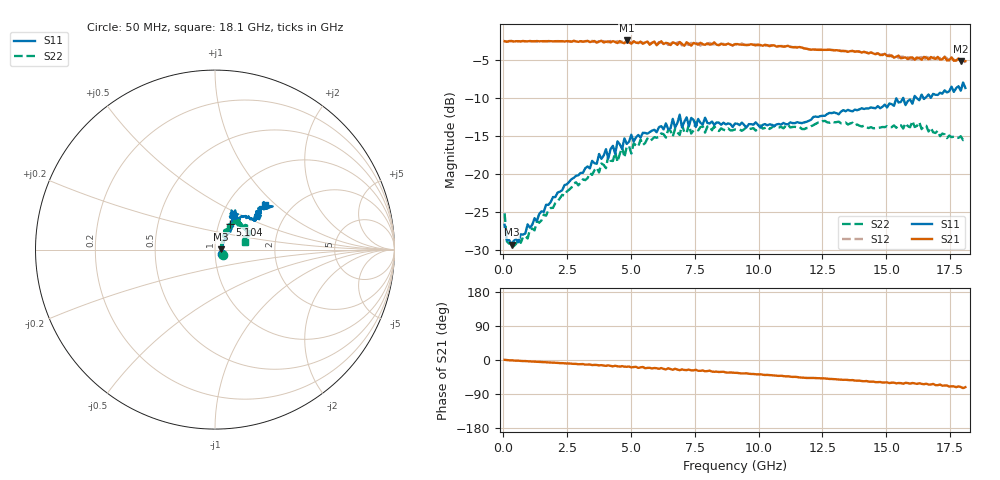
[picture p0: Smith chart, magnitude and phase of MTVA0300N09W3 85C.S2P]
! Network Analyzer HP8720D.06.14 Serial No. US36140669
!  7 Jul 2005  12:54:26
! Frequency  S11  S21  S12  S22
# HZ  S  DB R 50
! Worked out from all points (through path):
!   201 points, 50 MHz to 18.1 GHz, reference 50 ohm
!   highest |S21| = -2.37 dB at 4.833 GHz (marker M1); lowest = -5.1 dB at 17.92 GHz (marker M2)
!   group delay of S21, straight-line fit = 11.1 ps
!   lowest |S11| = -29.4 dB at 320.8 MHz (marker M3), VSWR 1.07, Z = 53.5 + j0.18 ohm
!   |S11| at or under -10 dB: start of sweep to 15.66 GHz; 15.67 GHz to 16.09 GHz (421.5 MHz wide, 2.65 % of centre); 16.2 GHz to 16.33 GHz (132.3 MHz wide, 0.814 % of centre)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
!   |S22| runs from -29.6 to -13.0 dB; largest |S21 - S12| = 0.042
!   S11 on the Smith chart (normalised r, x): 50 MHz: 1.08, -0.05; 5.104 GHz: 1.13, +0.33; 18.1 GHz: 1.48, +0.84
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5e7  -26.73 -33.5  -2.47 0.5  -2.50 0.5  -25.20 -31.9
1.4025e8  -28.69 -16.0  -2.55 -0.1  -2.54 -0.3  -28.94 -15.2
3.2075e8  -29.35 2.8  -2.44 -0.7  -2.48 -0.7  -28.93 1.2
9.525e8  -26.68 27.0  -2.50 -3.4  -2.44 -3.4  -28.54 28.9
3.1185e9  -19.85 51.5  -2.52 -10.7  -2.55 -11.2  -20.72 58.6
4.65275e9  -16.72 52.8  -2.65 -16.1  -2.52 -17.9  -16.43 63.0
4.743e9  -15.32 56.0  -2.74 -17.7  -2.61 -16.7  -17.83 59.6
4.83325e9  -16.04 61.2  -2.37 -17.8  -2.65 -18.3  -16.43 53.8
5.01375e9  -14.82 58.5  -2.80 -19.5  -2.75 -18.0  -17.33 56.8
5.104e9  -15.73 59.2  -2.47 -18.6  -2.61 -19.5  -15.96 56.2
6.09675e9  -13.82 58.2  -2.70 -23.2  -2.59 -23.0  -15.09 55.0
6.7285e9  -13.87 65.8  -2.73 -23.1  -3.02 -23.8  -14.02 49.5
6.909e9  -12.19 62.7  -2.57 -26.9  -2.64 -24.9  -14.87 49.7
6.99925e9  -13.86 62.6  -2.83 -24.8  -3.04 -27.0  -13.51 50.4
7.17975e9  -12.53 67.1  -2.61 -26.6  -2.87 -24.9  -14.60 46.2
7.54075e9  -13.79 59.9  -2.80 -25.8  -2.70 -29.0  -13.19 52.9
9.075e9  -13.36 62.1  -2.87 -33.8  -2.84 -33.9  -14.13 41.9
1.21435e10  -12.48 51.3  -3.56 -47.3  -3.51 -47.6  -13.56 39.3
1.512175e10  -10.71 36.3  -4.44 -60.9  -4.25 -60.4  -13.85 31.6
1.602425e10  -10.74 39.6  -4.62 -60.6  -4.91 -63.1  -13.03 26.9
1.79195e10  -9.02 39.5  -5.10 -71.3  -4.92 -71.6  -15.03 21.8
1.81e10  -8.64 41.7  -5.10 -71.6  -5.29 -72.6  -15.31 15.1
